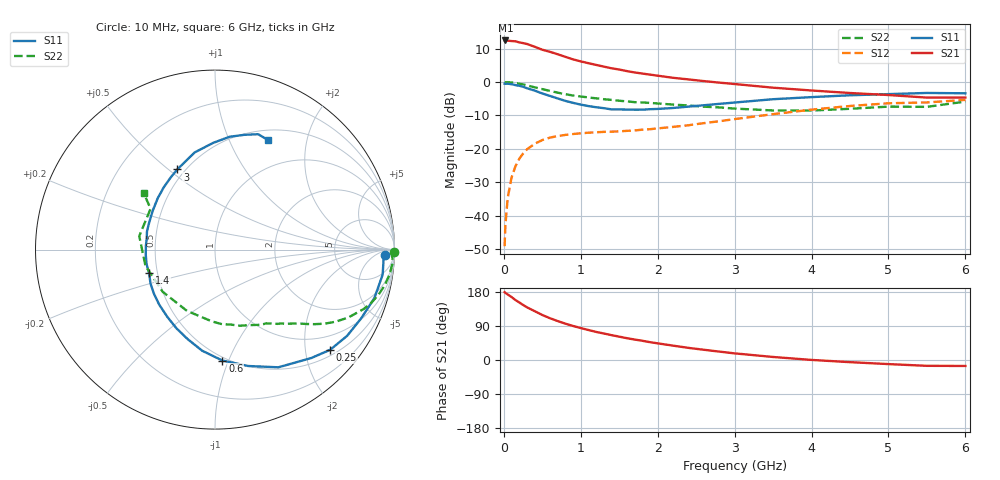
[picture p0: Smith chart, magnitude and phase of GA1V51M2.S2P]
! Infineon Technologies  Discrete & RF Semiconductors
! BF775
! Si NPN RF Bipolar Junction Transistor in SOT23
! VCE = 1.5 V  IC = 1.2 mA
! Common Emitter S-Parameters:  May  1996
# GHz  S  MA  R  50
!  f  S11  S21  S12  S22
! GHz  MAG  ANG  MAG  ANG  MAG  ANG  MAG  ANG
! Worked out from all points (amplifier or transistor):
!   36 points, 10 MHz to 6 GHz, reference 50 ohm
!   highest |S21| = 12.4 dB at 20 MHz (marker M1)
!   |S21| within 3 dB of that: start of sweep to 536 MHz
!   unconditionally stable (mu >= 1): 1.323 GHz to end of sweep
!   at 250 MHz: K = 0.22, MSG = 16.5 dB, |S12| = -21.4 dB
!   at 1.4 GHz: K = 1.05, MAG = 8.1 dB, |S12| = -14.8 dB
!   at 6 GHz: K = 1.06, MAG = -1.2 dB, |S12| = -5.3 dB
!   S11 on the Smith chart (normalised r, x): 10 MHz: 28, -15; 250 MHz: 0.63, -2.54; 600 MHz: 0.47, -0.95; 1.4 GHz: 0.45, -0.14; 3 GHz: 0.45, +0.54; 6 GHz: 0.62, +1.40
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0.01  0.9452 -1.7  4.119 179.0  0.0035 91.0  0.9983 -0.8
0.02  0.9408 -3.3  4.188 177.1  0.0072 89.5  0.9867 -1.5
0.05  0.9445 -8.5  4.155 173.0  0.0184 84.6  0.9928 -4.1
0.1  0.9282 -16.9  4.103 166.2  0.0371 79.5  0.9831 -8.0
0.15  0.9 -25.2  4.07 158.3  0.0545 74.2  0.9658 -12.0
0.25  0.8506 -41.0  3.823 145.3  0.0849 65.2  0.9208 -18.7
0.3  0.8079 -48.4  3.712 139.1  0.0982 61.3  0.892 -21.8
0.4  0.7448 -61.7  3.375 129.0  0.119 54.2  0.8336 -27.0
0.5  0.6743 -74.1  3.043 118.8  0.1355 48.5  0.7826 -30.9
0.6  0.6193 -86.2  2.831 110.2  0.1474 43.9  0.7364 -34.1
0.8  0.5219 -106.9  2.379 95.8  0.1618 37.4  0.6572 -39.1
0.9  0.488 -116.2  2.183 89.8  0.1666 35.4  0.6282 -41.0
1.1  0.4366 -135.4  1.914 79.1  0.1745 32.6  0.5876 -44.6
1.4  0.3898 -160.4  1.605 65.6  0.181 30.9  0.5404 -50.0
1.7  0.3855 176.8  1.391 54.0  0.1886 32.5  0.5 -55.3
2.2  0.4089 148.1  1.157 37.9  0.213 35.5  0.4597 -66.4
3  0.4935 115.2  0.933 17.5  0.2788 36.8  0.4005 -92.4
3.5  0.5533 101.8  0.823 8.0  0.3308 33.8  0.3755 -114.6
4.5  0.6336 82.7  0.685 -5.7  0.4383 22.5  0.3978 -166.9
5  0.6595 75.8  0.639 -10.8  0.4809 15.0  0.4287 169.9
5.5  0.6864 69.5  0.585 -15.4  0.4952 6.8  0.4251 147.6
6  0.6782 64.2  0.585 -15.7  0.5402 2.6  0.5097 141.4
